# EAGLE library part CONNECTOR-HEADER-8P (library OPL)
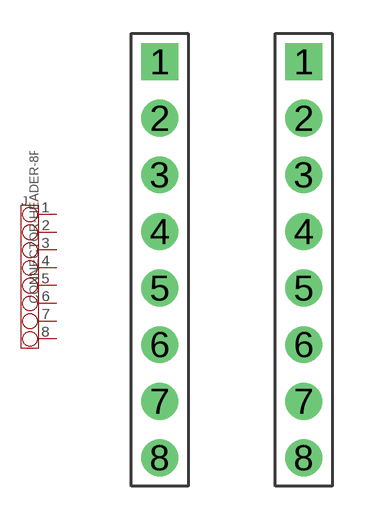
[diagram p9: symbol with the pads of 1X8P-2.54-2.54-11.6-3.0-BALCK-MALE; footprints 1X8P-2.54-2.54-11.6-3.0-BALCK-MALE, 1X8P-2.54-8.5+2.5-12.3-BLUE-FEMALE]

Designator prefix J

## CONNECTOR-HEADER-8P-3461050P1  [1X8P-2.54-2.54-11.6-3.0-BALCK-MALE]
1  1
2  2
3  3
4  4
5  5
6  6
7  7
8  8

## CONNECTOR-HEADER-8P-3461260P1  [1X8P-2.54-8.5+2.5-12.3-BLUE-FEMALE]
Pads as for 1X8P-2.54-2.54-11.6-3.0-BALCK-MALE

## CONNECTOR-HEADER-8P-3460290P1  [1X8P-2.54-8.5-BLACK-FEMALE]
Pads as for 1X8P-2.54-2.54-11.6-3.0-BALCK-MALE

## CONNECTOR-HEADER-8P-3460550P1  [1X8P-2.54-8.5-WHITE-FEMALE]
Pads as for 1X8P-2.54-2.54-11.6-3.0-BALCK-MALE

## CONNECTOR-HEADER-8P-3460590P1  [1X8P-2.54-8.5-YELLOW-FEMALE]
Pads as for 1X8P-2.54-2.54-11.6-3.0-BALCK-MALE

## Footprint 1X8P-2.54-2.54-11.6-3.0-BALCK-MALE (pad centres in mm)
drill 0.889 pad 1.651 square: 1 0,8.89
drill 0.889 pad 1.651: 2 0,6.35; 3 0,3.81; 4 0,1.27; 5 0,-1.27; 6 0,-3.81; 7 0,-6.35; 8 0,-8.89

## Footprint 1X8P-2.54-8.5+2.5-12.3-BLUE-FEMALE (pad centres in mm)
drill 0.889 pad 1.651 square: 1 0,8.89
drill 0.889 pad 1.651: 2 0,6.35; 3 0,3.81; 4 0,1.27; 5 0,-1.27; 6 0,-3.81; 7 0,-6.35; 8 0,-8.89

## Footprint 1X8P-2.54-8.5-BLACK-FEMALE (pad centres in mm)
drill 0.889 pad 1.651 square: 1 0,8.89
drill 0.889 pad 1.651: 2 0,6.35; 3 0,3.81; 4 0,1.27; 5 0,-1.27; 6 0,-3.81; 7 0,-6.35; 8 0,-8.89

## Footprint 1X8P-2.54-8.5-WHITE-FEMALE (pad centres in mm)
drill 0.889 pad 1.651 square: 1 0,8.89
drill 0.889 pad 1.651: 2 0,6.35; 3 0,3.81; 4 0,1.27; 5 0,-1.27; 6 0,-3.81; 7 0,-6.35; 8 0,-8.89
